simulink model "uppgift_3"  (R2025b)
settings: Solver=VariableStepAuto  StartTime=0.0  StopTime=10.0  RelTol=1e-3
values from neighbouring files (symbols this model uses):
  m_dot_end = 14*1e-3    (= 0.014)    [Lektion_2.m]
  m_dot_start = 12*1e-3    (= 0.012)    [Lektion_2.m]
  R = 280    [Lektion_2.m]
  T_i = 320    [Lektion_2.m]
  V_i = 2/1e3    (= 0.002)    [Lektion_2.m]
undefined symbols (not defined in the file or in its folder): p_im

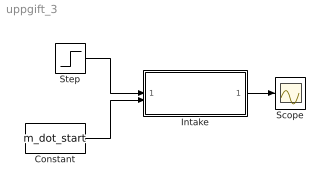
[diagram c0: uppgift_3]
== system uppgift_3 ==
  Constant : Constant  Value=m_dot_start
  Intake : Subsystem
  Scope : Scope
  Step : Step  Time=3  Before=m_dot_start  After=m_dot_end  SampleTime=0
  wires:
  Intake/1(p_im [Pa]) -> Scope/1
  Constant/1 -> Intake/2(m_ac [kg/s])
  Step/1 -> Intake/1(m_at [kg/s])

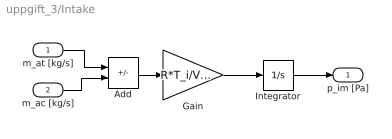
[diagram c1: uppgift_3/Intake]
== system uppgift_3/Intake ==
  m_at [kg/s] : Inport
  m_ac [kg/s] : Inport  Port=2
  Add : Sum  Inputs=+-
  Gain : Gain  Gain=R*T_i/V_i
  Integrator : Integrator  InitialCondition=p_im
  p_im [Pa] : Outport
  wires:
  Integrator/1 -> p_im [Pa]/1
  Gain/1 -> Integrator/1
  m_ac [kg/s]/1 -> Add/2
  m_at [kg/s]/1 -> Add/1
  Add/1 -> Gain/1
